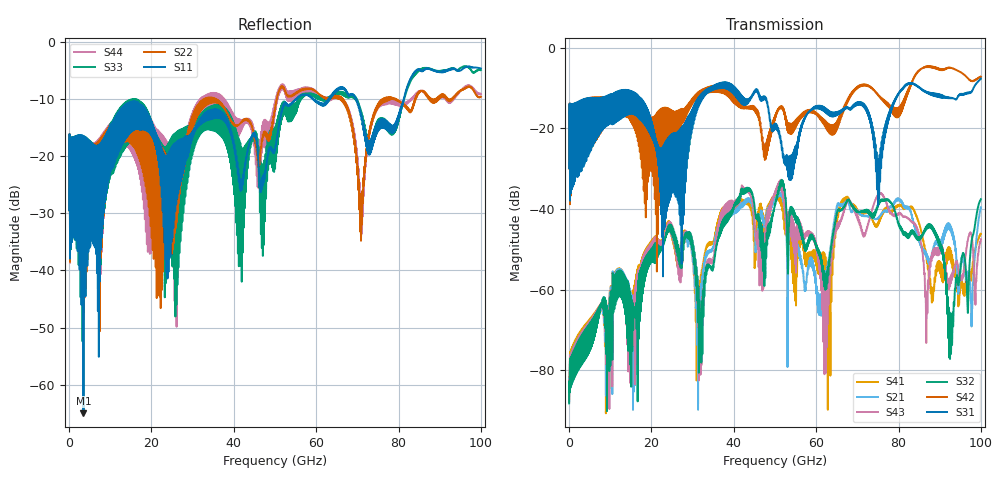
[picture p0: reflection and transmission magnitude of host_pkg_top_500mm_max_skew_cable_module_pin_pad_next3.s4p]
# Hz S RI R 50
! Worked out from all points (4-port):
!   10000 points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, 10 MHz to 100 GHz, reference 50 ohm
!   strongest paths, dB at 10 MHz, 25.01 GHz, 50.01 GHz, 75.01 GHz, 100 GHz:
!     S31: -29.9, -28.1, -18.9, -38.2, -7.6
!     S42: -29.9, -15.8, -16.8, -11.6, -7.2
!     S32: -88.3, -44.7, -38.8, -39.4, -37.6
!     S43: -87.9, -44.5, -35.6, -36.5, -47.5
!     S21: -87.7, -44.6, -37.5, -42.4, -39.5
!     S41: -87.3, -44.5, -37.0, -43.7, -46.2
!   lowest |S11| = -65.0 dB at 3.5 GHz (marker M1), VSWR 1.00, Z = 50 + j0.0494 ohm
!   |S11| at or under -10 dB: start of sweep to 55.26 GHz; 59.25 GHz to 63.15 GHz (3.898 GHz wide, 6.37 % of centre); 69.57 GHz to 81.29 GHz (11.72 GHz wide, 15.5 % of centre)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
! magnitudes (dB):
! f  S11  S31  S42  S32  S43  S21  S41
! 10 MHz  -29.5  -29.9  -29.9  -88.3  -87.9  -87.7  -87.3
! 3.5 GHz  -65.0  -22.3  -26.1  -71.1  -70.5  -70.4  -69.7
! 51.62 GHz  -12.2  -24.9  -14.6  -32.7  -33.4  -36.2  -38.5
! 60.99 GHz  -11.0  -14.4  -17.0  -52.3  -56.1  -66.4  -53.3
! 77.5 GHz  -15.4  -17.1  -14.1  -37.6  -40.1  -40.1  -40.3
! 92.74 GHz  -4.9  -12.4  -5.0  -75.6  -58.4  -44.3  -50.6
! 100 GHz  -4.7  -7.6  -7.2  -37.6  -47.5  -39.5  -46.2
